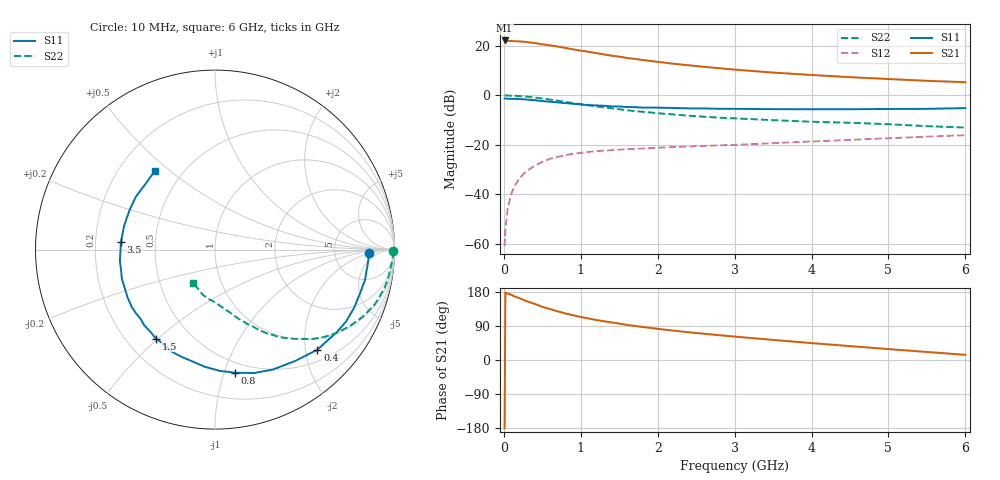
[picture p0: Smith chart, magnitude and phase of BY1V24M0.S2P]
! SIEMENS Small Signal Semiconductors
! BFY420
! Si NPN RF SIEGET Grounded Emitter Transistor in MICRO-X
! VCE = 1.25 V  IC = 4 mA
! Common Emitter S-Parameters:  October  1996
# GHz  S  MA  R  50
!  f  S11  S21  S12  S22
! GHz  MAG  ANG  MAG  ANG  MAG  ANG  MAG  ANG
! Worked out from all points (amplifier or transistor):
!   36 points, 10 MHz to 6 GHz, reference 50 ohm
!   highest |S21| = 22.2 dB at 10 MHz (marker M1)
!   |S21| within 3 dB of that: start of sweep to 794.3 MHz
!   unconditionally stable (mu >= 1): 3.297 GHz to end of sweep
!   at 250 MHz: K = 0.09, MSG = 26.8 dB, |S12| = -31.9 dB
!   at 1.4 GHz: K = 0.48, MSG = 19.1 dB, |S12| = -22.2 dB
!   at 6 GHz: K = 1.18, MAG = 8.2 dB, |S12| = -16.1 dB
!   S11 on the Smith chart (normalised r, x): 10 MHz: 13, -2; 400 MHz: 0.73, -2.25; 800 MHz: 0.41, -1.09; 1.5 GHz: 0.32, -0.49; 3.5 GHz: 0.31, +0.04; 6 GHz: 0.35, +0.44
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0.01  0.8595 -1.4  12.82 -180.0  0.0009 92.0  0.9904 -0.6
0.02  0.8574 -2.7  12.76 177.8  0.0019 84.3  0.9933 -1.3
0.05  0.8547 -5.6  12.5 175.2  0.0052 87.7  0.9897 -3.2
0.1  0.8524 -11.6  12.49 171.9  0.0106 84.4  0.9829 -6.5
0.15  0.8435 -17.1  12.34 166.7  0.0158 79.4  0.9771 -9.8
0.25  0.833 -28.8  12.14 158.9  0.0254 74.4  0.9535 -16.0
0.3  0.82 -34.0  11.9 154.9  0.0296 72.4  0.9408 -19.0
0.4  0.7979 -44.3  11.37 148.2  0.038 66.8  0.9026 -24.6
0.5  0.7652 -54.1  10.72 140.3  0.0452 61.4  0.8619 -29.8
0.6  0.7422 -64.1  10.24 134.5  0.0521 57.3  0.8208 -34.5
0.8  0.6952 -80.7  9.044 122.9  0.062 49.2  0.7359 -42.6
0.9  0.676 -87.8  8.463 118.0  0.0661 46.5  0.6972 -45.5
1.1  0.6345 -101.9  7.574 109.6  0.0721 41.8  0.6299 -51.5
1.3  0.6165 -113.7  6.714 102.3  0.0767 38.2  0.5714 -56.1
1.5  0.5953 -123.6  6.039 96.1  0.0799 35.5  0.5231 -60.2
1.8  0.5663 -137.2  5.179 87.3  0.0843 32.4  0.4659 -64.9
2.2  0.5554 -151.3  4.351 77.6  0.0901 30.1  0.4122 -70.6
2.8  0.5348 -168.2  3.528 65.5  0.0976 27.7  0.3532 -77.6
3.5  0.5259 175.5  2.879 53.0  0.1083 26.2  0.3153 -84.7
4.5  0.5243 155.4  2.327 36.7  0.1259 22.4  0.2793 -96.4
5.5  0.5335 136.0  1.963 21.2  0.1464 17.6  0.2386 -113.0
6  0.5517 127.6  1.843 13.7  0.1567 14.7  0.2235 -123.2
